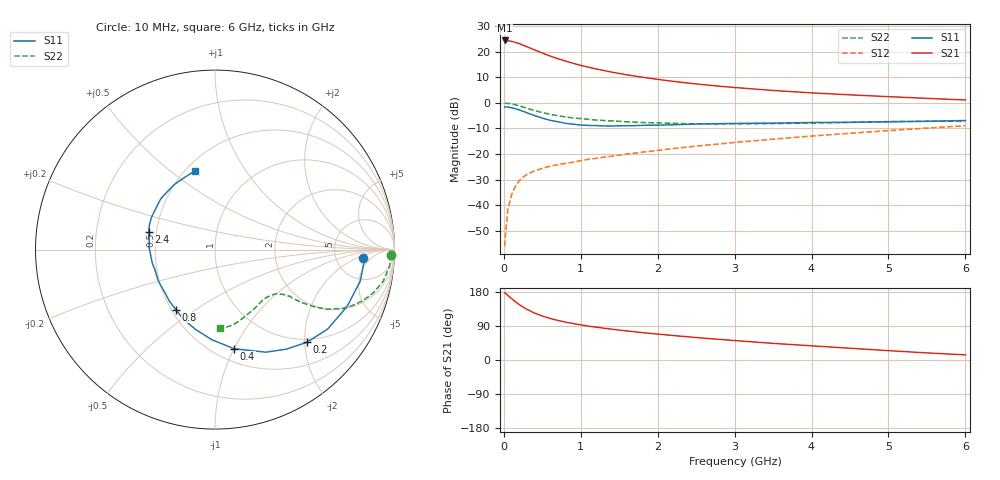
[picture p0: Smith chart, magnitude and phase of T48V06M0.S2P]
! Infineon Technologies  Discrete & RF Semiconductors
! BFR182T
! Si NPN RF Bipolar Junction Transistor in SC75
! VCE = 8 V  IC = 6 mA
! Common Emitter S-Parameters:  October  1999
# GHz  S  MA  R  50
!  f  S11  S21  S12  S22
! GHz  MAG  ANG  MAG  ANG  MAG  ANG  MAG  ANG
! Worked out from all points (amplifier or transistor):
!   36 points, 10 MHz to 6 GHz, reference 50 ohm
!   highest |S21| = 24.3 dB at 10 MHz (marker M1)
!   |S21| within 3 dB of that: start of sweep to 344.3 MHz
!   unconditionally stable (mu >= 1): 1.374 GHz to 4.096 GHz
!   at 250 MHz: K = 0.31, MSG = 25.8 dB, |S12| = -29.0 dB
!   at 1.4 GHz: K = 1.01, MAG = 15.9 dB, |S12| = -20.8 dB
!   at 6 GHz: K = 0.86, MSG = 5.0 dB, |S12| = -8.9 dB
!   lowest NFmin = 1.25 dB at 450 MHz
!   S11 on the Smith chart (normalised r, x): 10 MHz: 9.51, -2.91; 200 MHz: 0.93, -2.04; 400 MHz: 0.62, -1.00; 800 MHz: 0.53, -0.42; 2.4 GHz: 0.45, +0.11; 6 GHz: 0.56, +0.61
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0.01  0.8246 -3.4  16.49 177.0  0.0016 79.8  0.9799 -1.8
0.02  0.8348 -3.5  16.46 176.2  0.0025 95.8  0.9781 -2.1
0.05  0.8285 -12.2  16.35 170.7  0.0079 88.0  0.9772 -5.4
0.1  0.801 -23.4  15.85 162.2  0.0161 79.8  0.9542 -10.6
0.15  0.7682 -35.2  15.13 153.8  0.0234 73.5  0.915 -15.2
0.2  0.7269 -45.3  14.32 146.3  0.0305 69.9  0.8738 -18.9
0.25  0.6821 -54.4  13.35 139.7  0.0355 64.5  0.8273 -22.1
0.3  0.6381 -63.6  12.44 133.7  0.0401 62.5  0.7858 -24.6
0.4  0.5626 -79.1  10.78 123.7  0.0473 57.8  0.7062 -28.1
0.5  0.5033 -91.8  9.36 116.1  0.0527 55.9  0.6469 -29.7
0.6  0.4574 -103.8  8.206 109.7  0.058 54.6  0.5984 -30.8
0.7  0.4275 -113.8  7.292 104.5  0.0622 54.4  0.5608 -31.4
0.8  0.3995 -123.1  6.544 100.0  0.066 54.6  0.5321 -31.8
0.9  0.383 -131.9  5.908 96.2  0.0697 55.2  0.5079 -32.0
1.1  0.3629 -146.3  4.961 89.4  0.0792 56.1  0.4763 -32.6
1.6  0.3587 -171.9  3.523 76.6  0.1001 58.9  0.4269 -35.0
2.2  0.3741 169.5  2.627 64.6  0.1282 60.8  0.3996 -40.3
2.4  0.3816 164.9  2.426 61.1  0.138 61.5  0.3924 -42.5
3.5  0.4024 144.4  1.743 43.9  0.1953 60.9  0.3949 -55.8
4.5  0.4176 129.9  1.433 31.0  0.255 57.9  0.4157 -69.5
5.5  0.4372 112.4  1.223 18.7  0.3219 53.5  0.4364 -81.7
6  0.4524 104.3  1.138 13.5  0.3579 50.3  0.4365 -86.7
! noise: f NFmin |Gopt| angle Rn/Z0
0.45  1.25  0.25  39  0.3
0.9  1.4  0.25  78  0.23
1.8  1.95  0.21  151  0.2
